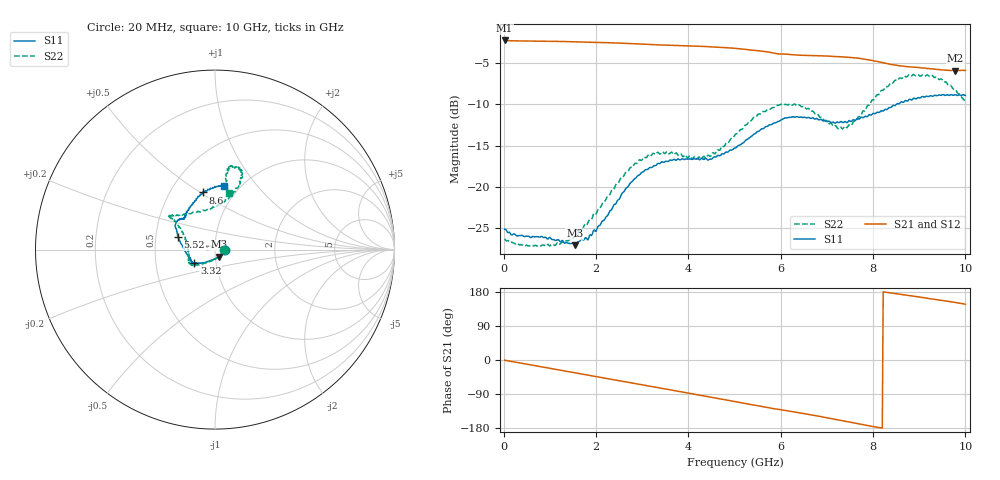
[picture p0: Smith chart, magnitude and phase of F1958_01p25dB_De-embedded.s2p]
! Integrated Device Technology
! Corporate Headquarters
! 6024 Silver Creek Valley Road
! San Jose, CA 95138  USA
! Phone:  1-408-284-8200
! Toll Free:  1-800-223-1366
! Webpage:  http://www.idt.com/
! Timing and RF Division
! 515 Groton Road, Suite 102
! Westford, MA 01886-6024
! Device:  F1958
! Description: 7-bit 0.25 dB Digital Step Attenuator
! Frequency:  0.001 -  6.000 GHz
! Package:  4x4 mm Thin QFN Plastic Package: 24 pin
! Ports:  2 RF, 12 DC
!  Pin  1  = D0
!  Pin  2  = VDD
!  Pin  3  = VMODE
!  Pin  4  = GND
!  Pin  5  = RF1  =  Port 1
!  Pin  6  = GND
!  Pin  7  = GND
!  Pin  8  = GND
!  Pin  9  = GND
!  Pin 10  = GND
!  Pin 11  = GND
!  Pin 12  = GND
!  Pin 13  = GND
!  Pin 14  = RF2  =  Port 2
!  Pin 15  = GND
!  Pin 16  = LE
!  Pin 17  = CLK
!  Pin 18  = DATA
!  Pin 19  = D6
!  Pin 20  = D5
!  Pin 21  = D4
!  Pin 22  = D3
!  Pin 23  = D2
!  Pin 24  = D1
! State:  5
! Atten State:  1.25 dB
! Voltage:  +3.30 Volts
! Current:  0.257 mA
! Data:  The device was measured on a F1958 evaluation board which has
!  individual transmission lines to the RF pins.  Data was collected
!  using a calibrated network analyzer.  The evaluation board was
!  de-embedded using Automatic Fixture Removal (AFR).
!  The reference plane is the edge of the package pin.
! Misc:
!  Action Tracker AT0419
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# GHz S dB R 50
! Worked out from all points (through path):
!   500 points, 20 MHz to 10 GHz, reference 50 ohm
!   highest |S21| = -2.29 dB at 20 MHz (marker M1); lowest = -5.9 dB at 9.78 GHz (marker M2)
!   group delay of S21, straight-line fit = 59.9 ps
!   lowest |S11| = -27.1 dB at 1.54 GHz (marker M3), VSWR 1.09, Z = 52 - j4.08 ohm
!   |S11| at or under -10 dB: start of sweep to 8.508 GHz
!   |S22| runs from -27.2 to -6.4 dB; largest |S21 - S12| = 0.0019
!   S11 on the Smith chart (normalised r, x): 20 MHz: 1.12, -0.01; 3.32 GHz: 0.79, -0.12; 5.52 GHz: 0.65, +0.10; 8.6 GHz: 0.72, +0.51; 10 GHz: 0.85, +0.69
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0.02  -25.13 -2.4  -2.29 -0.6  -2.29 -0.6  -26.29 -3.2
0.76  -26.06 -17.0  -2.38 -16.6  -2.37 -16.6  -27.06 -28.0
1.22  -26.61 -41.4  -2.41 -26.7  -2.41 -26.7  -26.91 -59.5
1.54  -27.07 -62.1  -2.45 -33.7  -2.45 -33.7  -25.87 -83.0
1.7  -26.33 -73.9  -2.47 -37.1  -2.47 -37.1  -25.23 -94.5
2.02  -25.09 -99.6  -2.52 -44.1  -2.51 -44.1  -23.07 -113.2
2.72  -19.73 -134.0  -2.66 -59.5  -2.65 -59.5  -17.86 -138.7
3.32  -17.26 -147.2  -2.82 -72.5  -2.82 -72.6  -15.88 -150.0
3.36  -17.18 -147.0  -2.83 -73.4  -2.83 -73.5  -15.92 -149.2
4.32  -16.65 -158.1  -3.01 -94.3  -3.03 -94.4  -16.34 179.5
5.02  -15.31 179.2  -3.25 -110.0  -3.26 -110.0  -13.63 151.8
5.52  -13.27 161.3  -3.54 -121.1  -3.55 -121.1  -11.18 144.9
6  -11.94 150.5  -3.93 -131.0  -3.94 -131.0  -10.02 143.6
6.68  -11.66 139.4  -4.12 -145.1  -4.14 -145.0  -10.84 137.4
7.2  -12.22 135.1  -4.24 -156.9  -4.25 -156.8  -12.64 113.7
7.4  -12.10 133.5  -4.31 -161.6  -4.31 -161.5  -12.68 99.6
7.92  -11.26 122.2  -4.65 -173.8  -4.65 -173.8  -10.11 74.2
8.34  -10.44 110.3  -5.13 177.6  -5.13 177.6  -7.76 69.1
8.6  -9.75 102.0  -5.37 173.1  -5.37 173.2  -6.85 71.7
9.26  -8.99 86.6  -5.72 161.3  -5.73 161.3  -6.54 78.9
9.78  -8.84 81.9  -5.94 151.8  -5.96 151.8  -8.21 80.3
10  -8.93 82.2  -5.91 147.1  -5.94 147.2  -9.70 76.2
